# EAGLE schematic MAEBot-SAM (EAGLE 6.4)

## Sheet 1 of 4: SAMA5
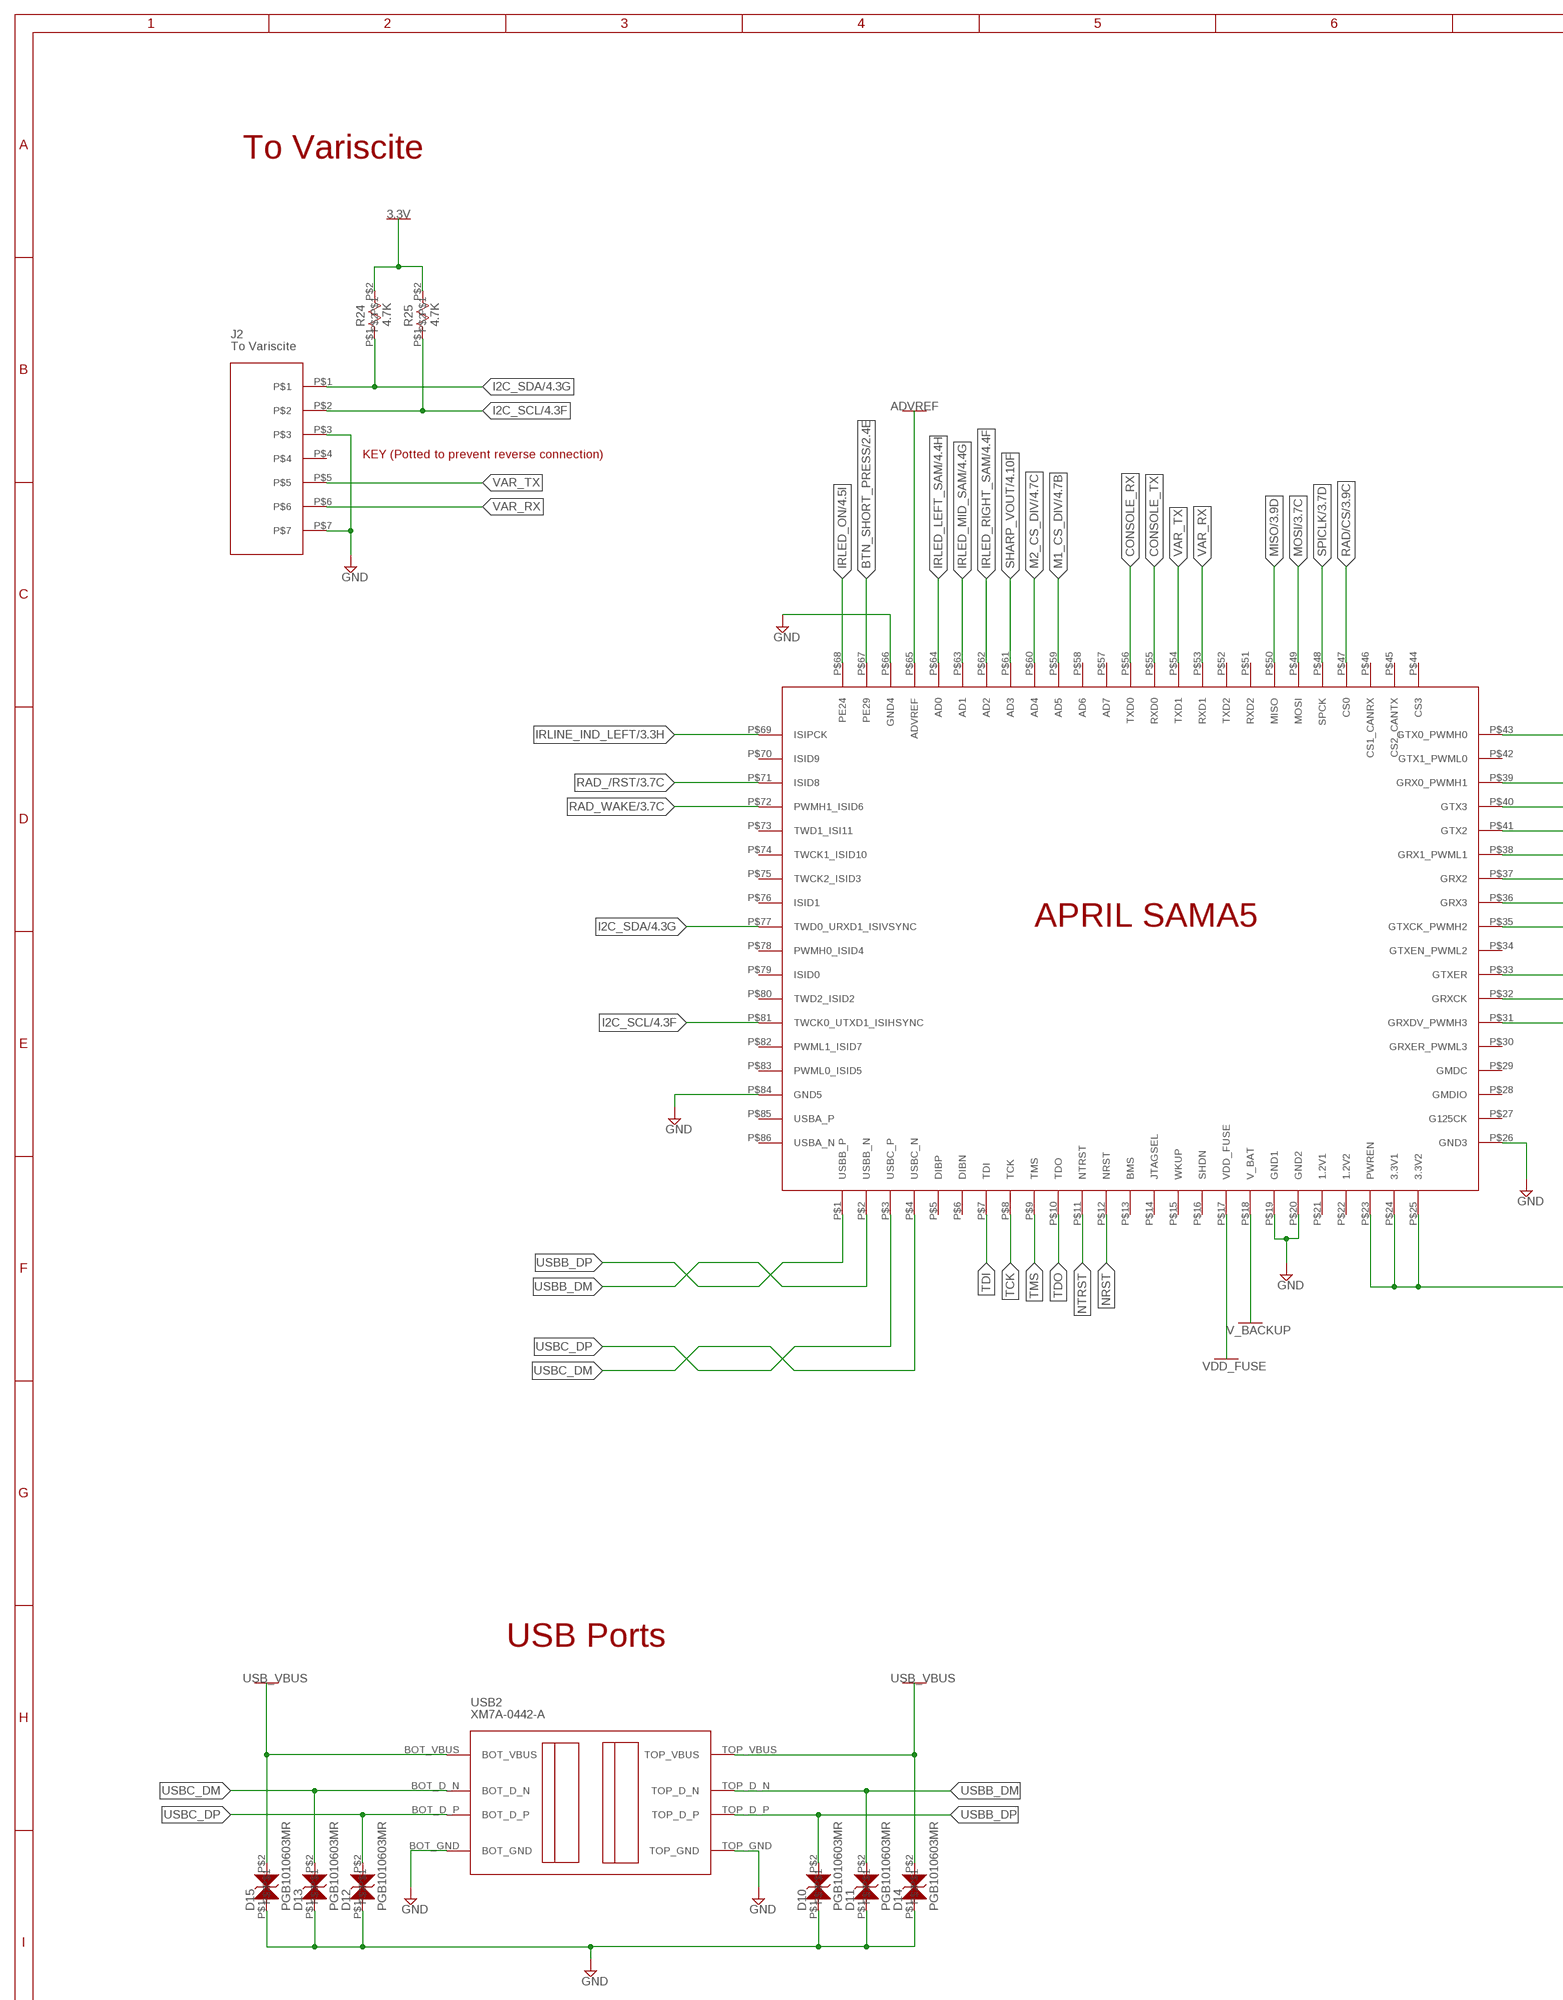
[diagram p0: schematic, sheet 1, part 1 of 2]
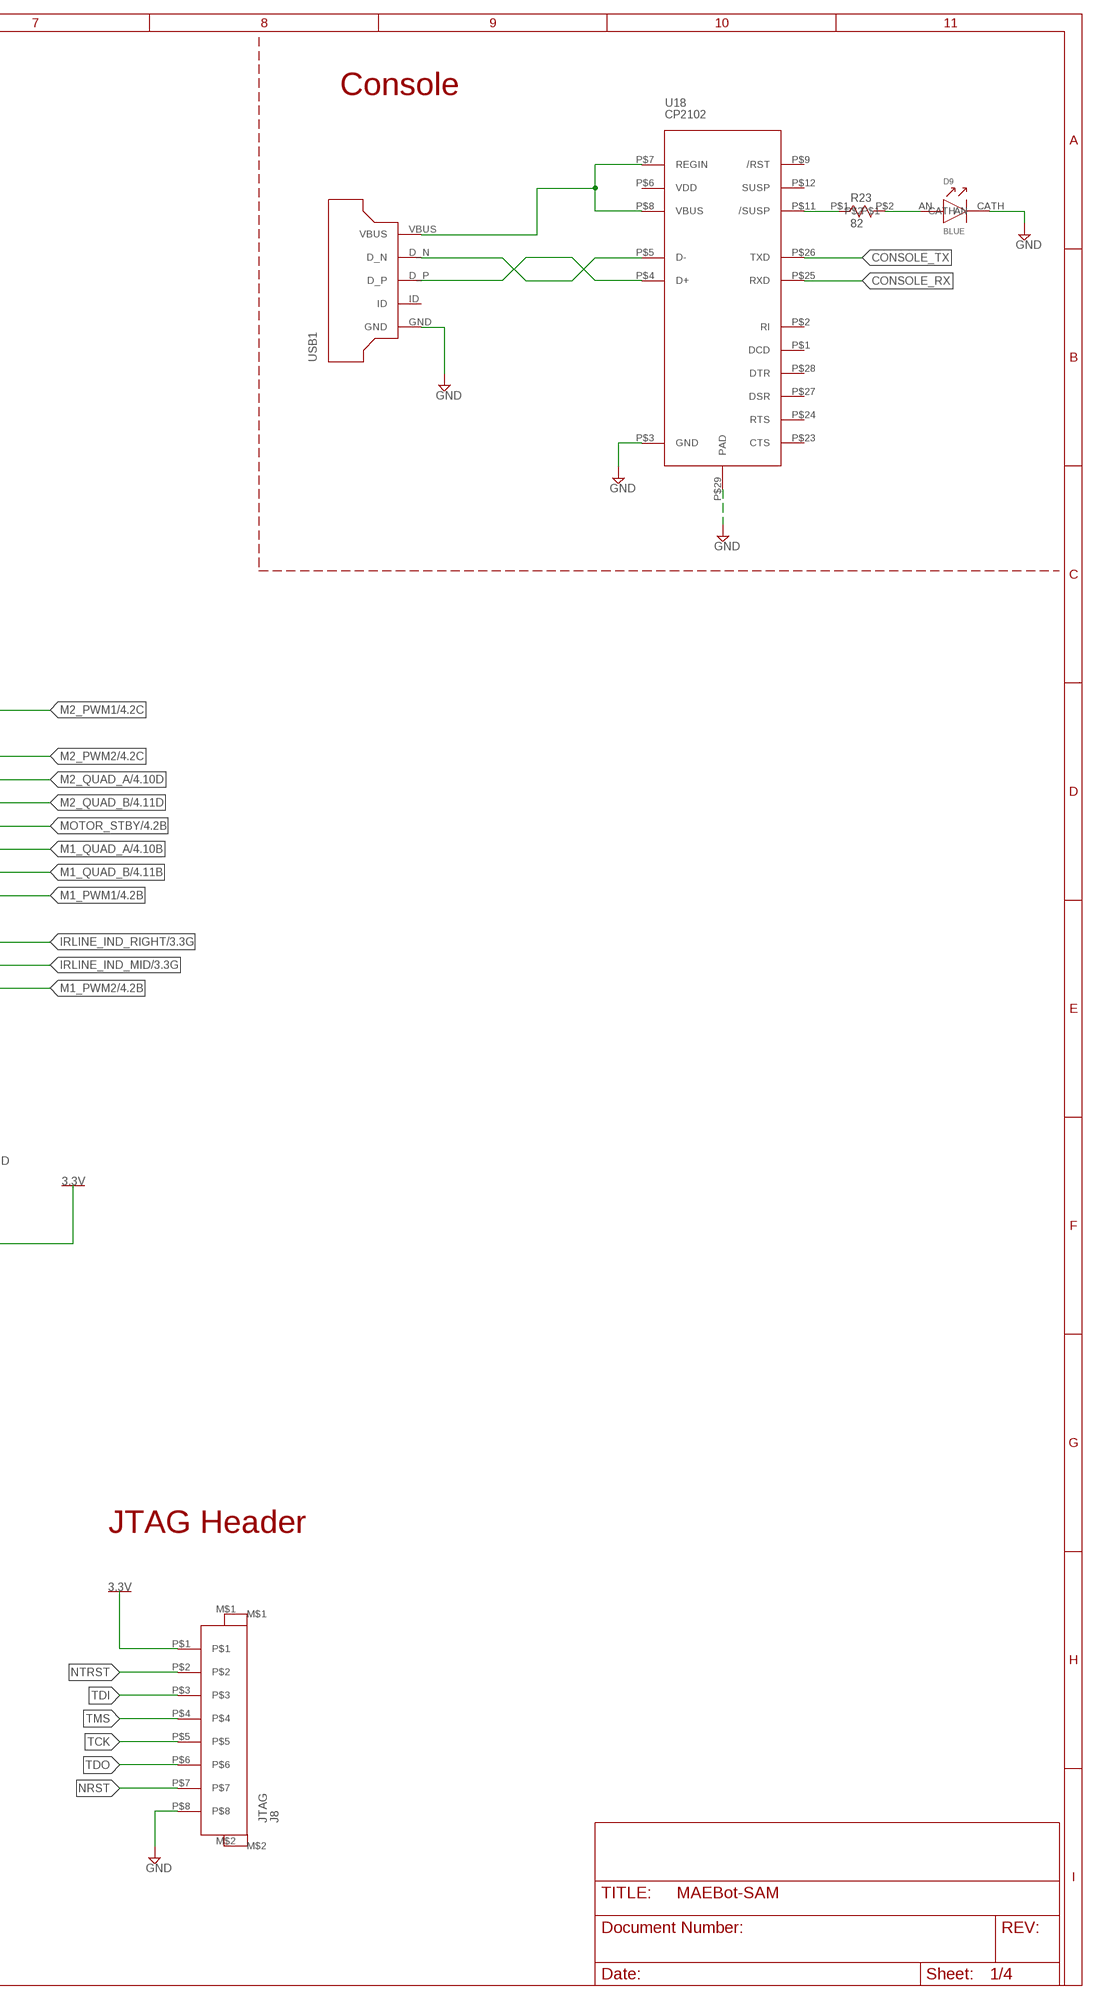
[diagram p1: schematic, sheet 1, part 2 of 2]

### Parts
D9  BLUE  LED0603  [D0603]
D10  PGB1010603MR  TVS0603  [SM0603]
D11  PGB1010603MR  TVS0603  [SM0603]
D12  PGB1010603MR  TVS0603  [SM0603]
D13  PGB1010603MR  TVS0603  [SM0603]
D14  PGB1010603MR  TVS0603  [SM0603]
D15  PGB1010603MR  TVS0603  [SM0603]
J2  To Variscite  J7X1  [J7X1]
J8  JTAG  PICOBLADE-8  [PICO-8]
R23  82  R0402  [R0402]
R24  4.7K  R0402  [R0402]
R25  4.7K  R0402  [R0402]
SAMA1  SAMA5_CARRIER  [SAMA5_CARRIER]
U18  CP2102  [28QFN-5MM]
USB1  USB_MINI_A  [USB_MINI_A]
USB2  XM7A-0442-A  [XM7A-0442-A]

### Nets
3.3V: J8.P$1 R24.P$2 R25.P$2 SAMA1.P$23(PWREN) SAMA1.P$24(3.3V1) SAMA1.P$25(3.3V2) ; also sheet 2,3,4
ADVREF: SAMA1.P$65(ADVREF) ; also sheet 2,4
BTN_SHORT_PRESS: SAMA1.P$67(PE29) ; also sheet 2,3
CONSOLE_/SUSP: R23.P$1 U18.P$11(/SUSP)
CONSOLE_DM: U18.P$5(D-) USB1.D_N
CONSOLE_DP: U18.P$4(D+) USB1.D_P
CONSOLE_LED: D9.AN R23.P$2
CONSOLE_RX: SAMA1.P$56(TXD0) U18.P$25(RXD)
CONSOLE_TX: SAMA1.P$55(RXD0) U18.P$26(TXD)
CONSOLE_VBUS: U18.P$7(REGIN) U18.P$8(VBUS) USB1.VBUS
GND: D9.CATH D10.P$1 D11.P$1 D12.P$1 D13.P$1 D14.P$1 D15.P$1 J2.P$3 J2.P$7 J8.P$8 SAMA1.P$19(GND1) SAMA1.P$20(GND2) SAMA1.P$26(GND3) SAMA1.P$66(GND4) SAMA1.P$84(GND5) U18.P$3(GND) U18.P$29(PAD) USB1.GND USB2.BOT_GND USB2.TOP_GND ; also sheet 2,3,4
I2C_SCL: J2.P$2 R25.P$1 SAMA1.P$81(TWCK0_UTXD1_ISIHSYNC) ; also sheet 4
I2C_SDA: J2.P$1 R24.P$1 SAMA1.P$77(TWD0_URXD1_ISIVSYNC) ; also sheet 4
IRLED_LEFT_SAM: SAMA1.P$64(AD0) ; also sheet 4
IRLED_MID_SAM: SAMA1.P$63(AD1) ; also sheet 4
IRLED_ON: SAMA1.P$68(PE24) ; also sheet 4
IRLED_RIGHT_SAM: SAMA1.P$62(AD2) ; also sheet 4
IRLINE_IND_LEFT: SAMA1.P$69(ISIPCK) ; also sheet 3
IRLINE_IND_MID: SAMA1.P$32(GRXCK) ; also sheet 3
IRLINE_IND_RIGHT: SAMA1.P$33(GTXER) ; also sheet 3
M1_CS_DIV: SAMA1.P$59(AD5) ; also sheet 4
M1_PWM1: SAMA1.P$35(GTXCK_PWMH2) ; also sheet 4
M1_PWM2: SAMA1.P$31(GRXDV_PWMH3) ; also sheet 4
M1_QUAD_A: SAMA1.P$37(GRX2) ; also sheet 4
M1_QUAD_B: SAMA1.P$36(GRX3) ; also sheet 4
M2_CS_DIV: SAMA1.P$60(AD4) ; also sheet 4
M2_PWM1: SAMA1.P$43(GTX0_PWMH0) ; also sheet 4
M2_PWM2: SAMA1.P$39(GRX0_PWMH1) ; also sheet 4
M2_QUAD_A: SAMA1.P$40(GTX3) ; also sheet 4
M2_QUAD_B: SAMA1.P$41(GTX2) ; also sheet 4
MISO: SAMA1.P$50(MISO) ; also sheet 3
MOSI: SAMA1.P$49(MOSI) ; also sheet 3
MOTOR_STBY: SAMA1.P$38(GRX1_PWML1) ; also sheet 4
NRST: J8.P$7 SAMA1.P$12(NRST)
NTRST: J8.P$2 SAMA1.P$11(NTRST)
RAD/CS: SAMA1.P$47(CS0) ; also sheet 3
RAD_/RST: SAMA1.P$71(ISID8) ; also sheet 3
RAD_WAKE: SAMA1.P$72(PWMH1_ISID6) ; also sheet 3
SHARP_VOUT: SAMA1.P$61(AD3) ; also sheet 4
SPICLK: SAMA1.P$48(SPCK) ; also sheet 3
TCK: J8.P$5 SAMA1.P$8(TCK)
TDI: J8.P$3 SAMA1.P$7(TDI)
TDO: J8.P$6 SAMA1.P$10(TDO)
TMS: J8.P$4 SAMA1.P$9(TMS)
USB_VBUS: D14.P$2 D15.P$2 USB2.BOT_VBUS USB2.TOP_VBUS ; also sheet 2
USBB_DM: D11.P$2 SAMA1.P$2(USBB_N) USB2.TOP_D_N
USBB_DP: D10.P$2 SAMA1.P$1(USBB_P) USB2.TOP_D_P
USBC_DM: D13.P$2 SAMA1.P$4(USBC_N) USB2.BOT_D_N
USBC_DP: D12.P$2 SAMA1.P$3(USBC_P) USB2.BOT_D_P
V_BACKUP: SAMA1.P$18(V_BAT) ; also sheet 2,3
VAR_RX: J2.P$6 SAMA1.P$53(RXD1)
VAR_TX: J2.P$5 SAMA1.P$54(TXD1)
VDD_FUSE: SAMA1.P$17(VDD_FUSE) ; also sheet 2
Unconnected: J2.P$4 J8.M$1 J8.M$2 SAMA1.P$5(DIBP) SAMA1.P$6(DIBN) SAMA1.P$13(BMS) SAMA1.P$14(JTAGSEL) SAMA1.P$15(WKUP) SAMA1.P$16(SHDN) SAMA1.P$21(1.2V1) SAMA1.P$22(1.2V2) SAMA1.P$27(G125CK) SAMA1.P$28(GMDIO) SAMA1.P$29(GMDC) SAMA1.P$30(GRXER_PWML3) SAMA1.P$34(GTXEN_PWML2) SAMA1.P$42(GTX1_PWML0) SAMA1.P$44(CS3) SAMA1.P$45(CS2_CANTX) SAMA1.P$46(CS1_CANRX) SAMA1.P$51(RXD2) SAMA1.P$52(TXD2) SAMA1.P$57(AD7) SAMA1.P$58(AD6) SAMA1.P$70(ISID9) SAMA1.P$73(TWD1_ISI11) SAMA1.P$74(TWCK1_ISID10) SAMA1.P$75(TWCK2_ISID3) SAMA1.P$76(ISID1) SAMA1.P$78(PWMH0_ISID4) SAMA1.P$79(ISID0) SAMA1.P$80(TWD2_ISID2) SAMA1.P$82(PWML1_ISID7) SAMA1.P$83(PWML0_ISID5) SAMA1.P$85(USBA_P) SAMA1.P$86(USBA_N) U18.P$1(DCD) U18.P$2(RI) U18.P$9(/RST) U18.P$12(SUSP) U18.P$23(CTS) U18.P$24(RTS) U18.P$27(DSR) U18.P$28(DTR) USB1.ID

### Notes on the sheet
- Console
- To Variscite
- KEY (Potted to prevent reverse connection)
- APRIL SAMA5
- JTAG Header
- USB Ports

## Sheet 2 of 4: Power
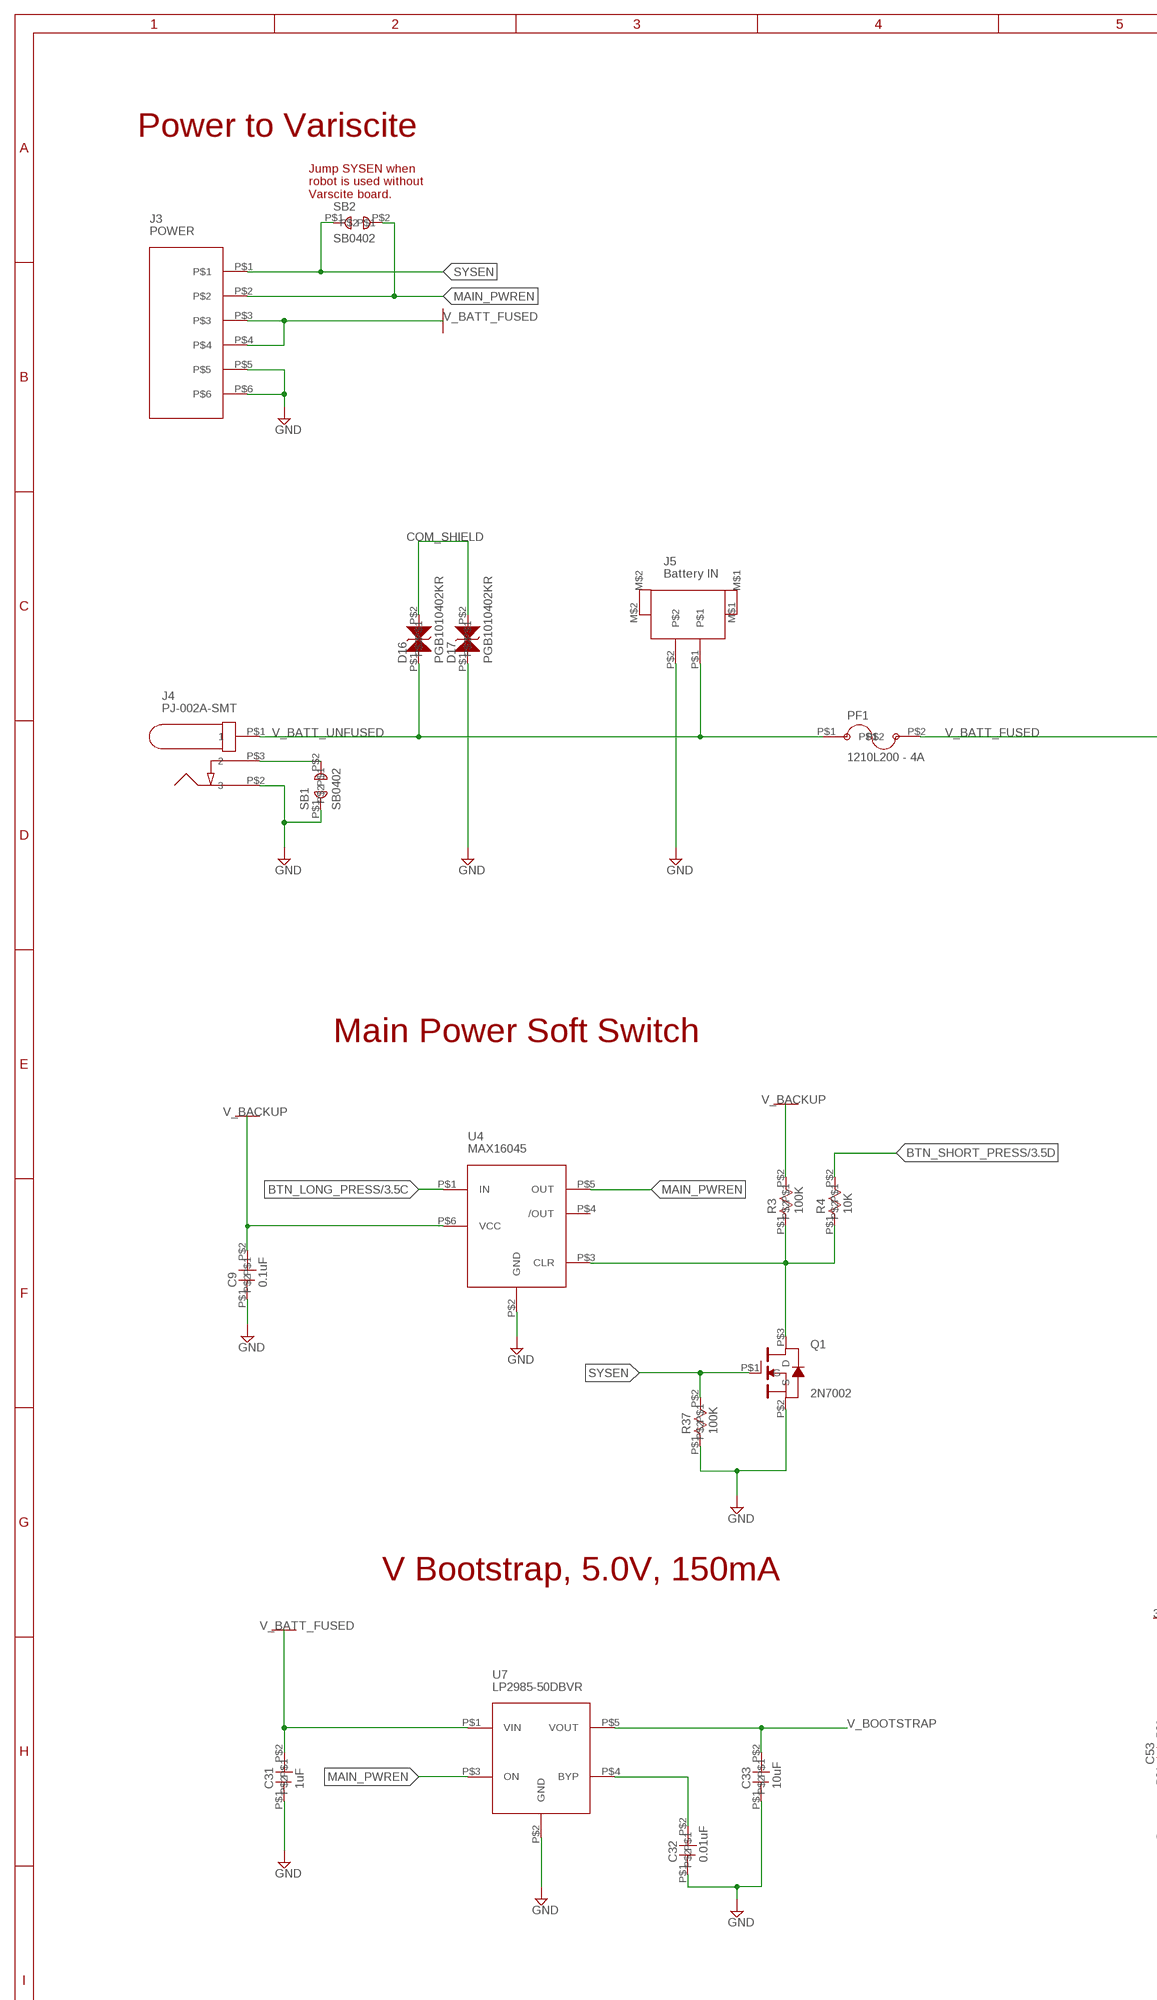
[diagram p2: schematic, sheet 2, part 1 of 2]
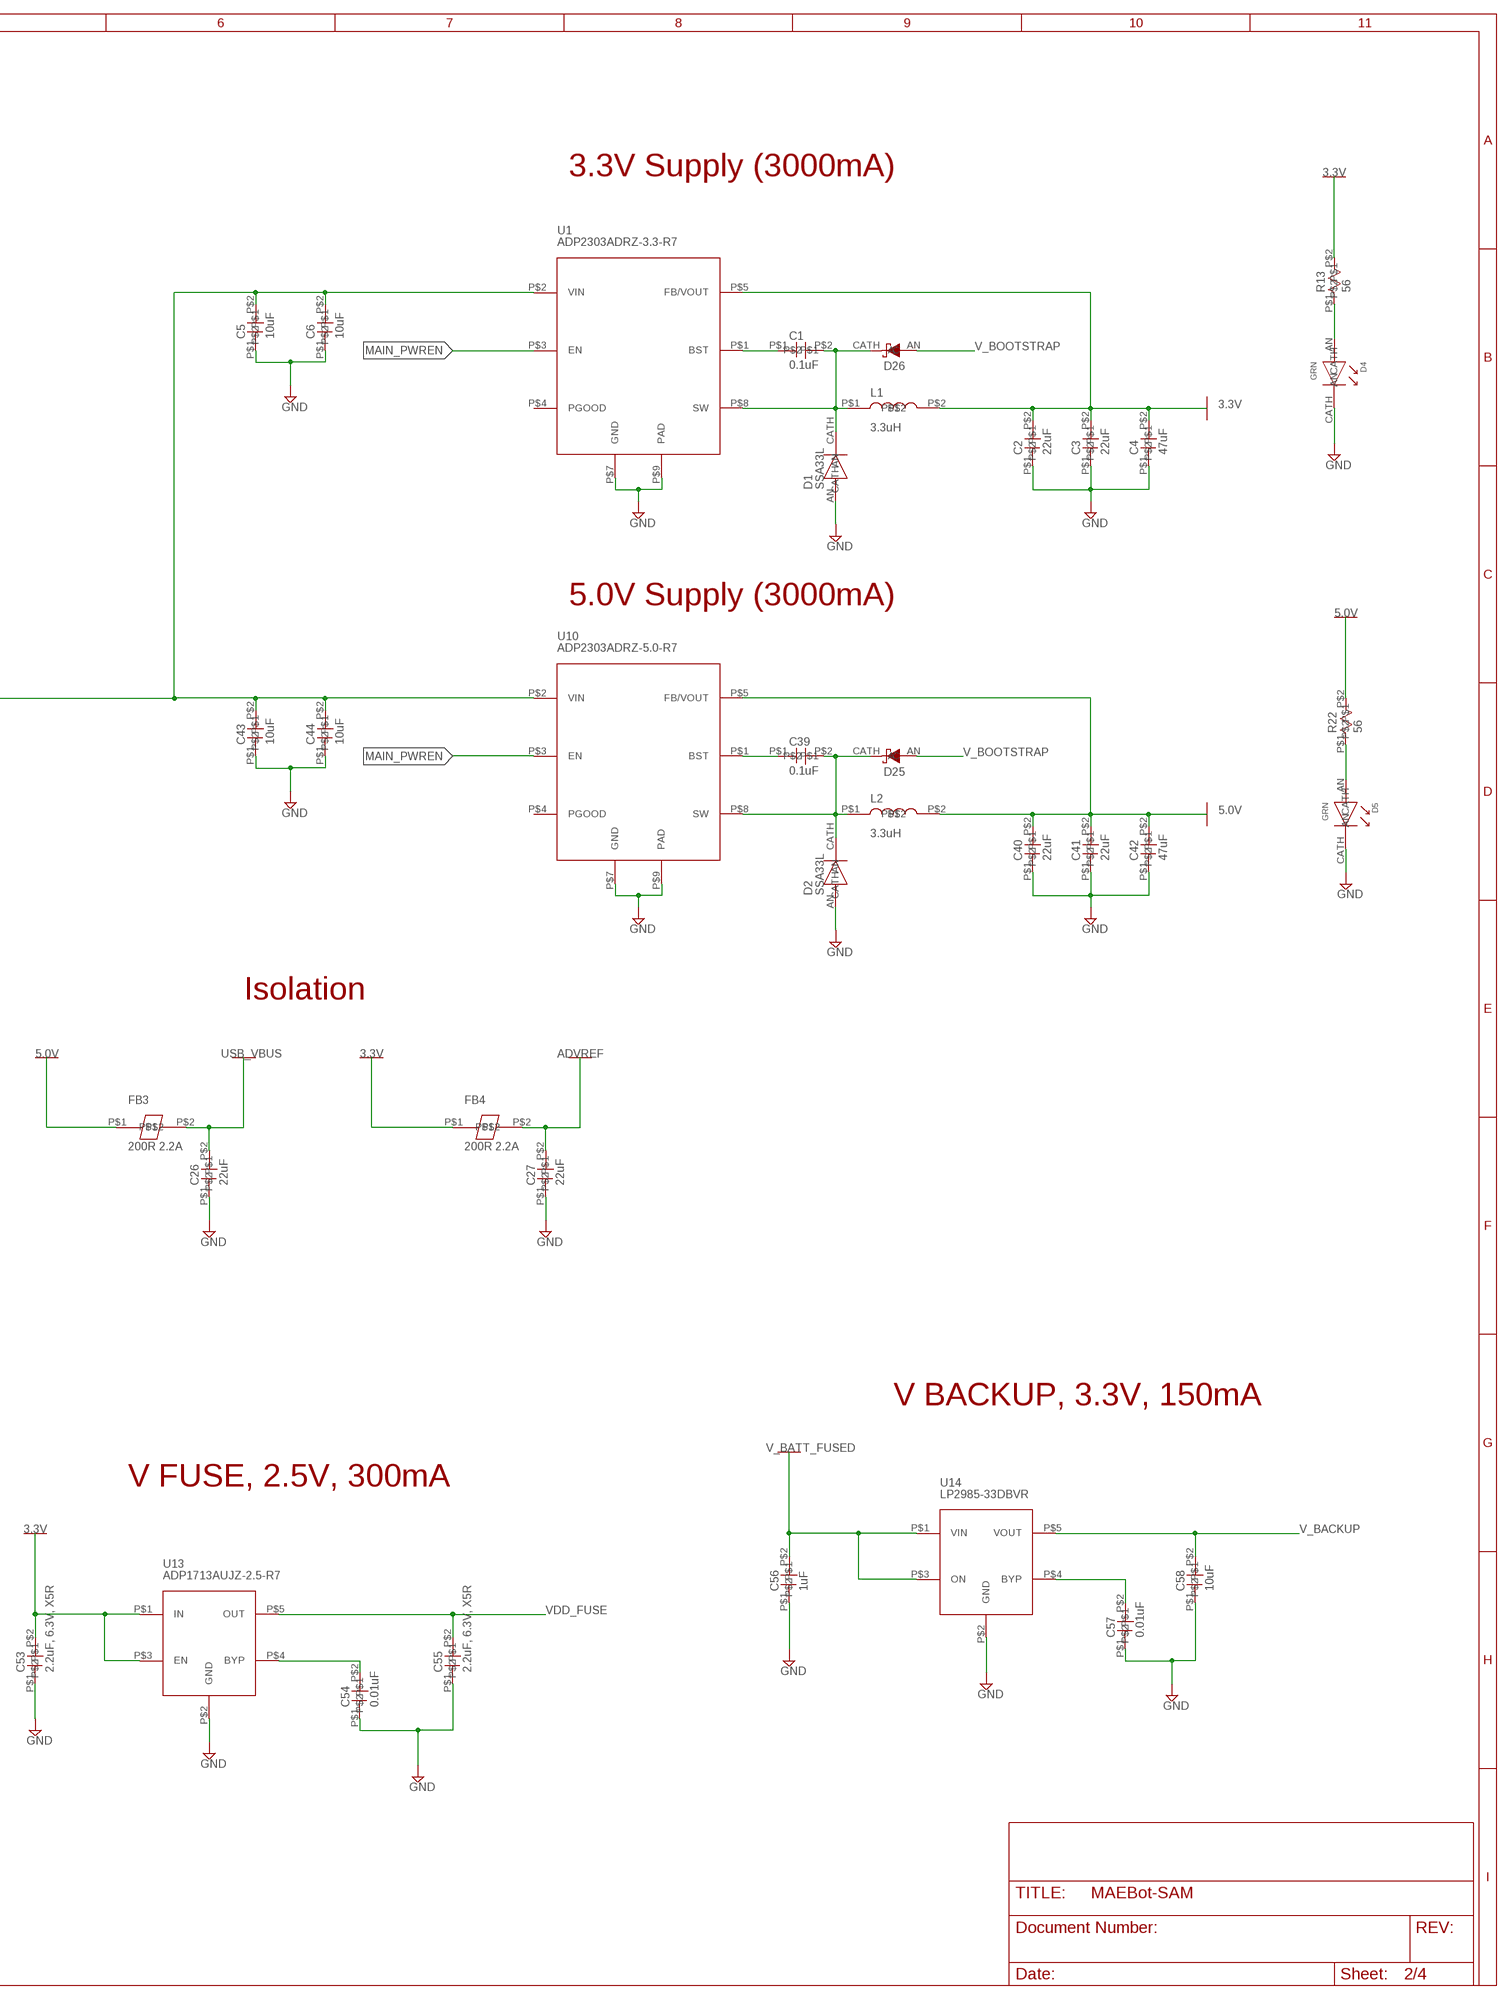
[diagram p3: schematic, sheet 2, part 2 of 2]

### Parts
C1  0.1uF  C0402  [R0402]
C2  22uF  C0603  [SM0603]
C3  22uF  C0603  [SM0603]
C4  47uF  C0805  [SM0805]
C5  10uF  C0603  [SM0603]
C6  10uF  C0603  [SM0603]
C9  0.1uF  C0402  [R0402]
C26  22uF  C0603  [SM0603]
C27  22uF  C0603  [SM0603]
C31  1uF  C0402  [R0402]
C32  0.01uF  C0402  [R0402]
C33  10uF  C0805  [SM0805]
C39  0.1uF  C0402  [R0402]
C40  22uF  C0603  [SM0603]
C41  22uF  C0603  [SM0603]
C42  47uF  C0805  [SM0805]
C43  10uF  C0603  [SM0603]
C44  10uF  C0603  [SM0603]
C53  2.2uF, 6.3V, X5R  C0402  [R0402]
C54  0.01uF  C0402  [R0402]
C55  2.2uF, 6.3V, X5R  C0805  [SM0805]
C56  1uF  C0402  [R0402]
C57  0.01uF  C0402  [R0402]
C58  10uF  C0805  [SM0805]
D1  SSA33L  [SSA33L]
D2  SSA33L  [SSA33L]
D4  GRN  LED0603  [D0603]
D5  GRN  LED0603  [D0603]
D16  PGB1010402KR  TVS0402  [R0402]
D17  PGB1010402KR  TVS0402  [R0402]
D25  DS0603  [D0603]
D26  DS0603  [D0603]
FB3  200R 2.2A  FB0603  [SM0603]
FB4  200R 2.2A  FB0603  [SM0603]
J3  POWER  J6X1  [J6X1]
J4  PJ-002A-SMT  [PJ-002A-SMT]
J5  Battery IN  PICOBLADE-2  [PICO-2]
L1  3.3uH  VLF10040  [VLF10040_SERIES]
L2  3.3uH  VLF10040  [VLF10040_SERIES]
PF1  1210L200 - 4A  1210L  [1210L_SERIES]
Q1  2N7002  [SOT23]
R3  100K  R0402  [R0402]
R4  10K  R0402  [R0402]
R13  56  R0402  [R0402]
R22  56  R0402  [R0402]
R37  100K  R0402  [R0402]
SB1  SB0402  [R0402]
SB2  SB0402  [R0402]
U1  ADP2303ADRZ-3.3-R7  [RD-8-1]
U4  MAX16045  [90-0240]
U7  LP2985-50DBVR  LP2985  [R-PDS0-G5_(SOT23-5)]
U10  ADP2303ADRZ-5.0-R7  [RD-8-1]
U13  ADP1713AUJZ-2.5-R7  ADP1713  [ADP171X_(SOT23-5)]
U14  LP2985-33DBVR  LP2985  [R-PDS0-G5_(SOT23-5)]

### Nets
3.3V: C2.P$2 C3.P$2 C4.P$2 C53.P$2 FB4.P$1 L1.P$2 R13.P$2 U1.P$5(FB/VOUT) U13.P$1(IN) U13.P$3(EN) ; also sheet 1,3,4
3.3V_BYP: C57.P$2 U14.P$4(BYP)
5.0V: C40.P$2 C41.P$2 C42.P$2 FB3.P$1 L2.P$2 R22.P$2 U10.P$5(FB/VOUT) ; also sheet 4
5.0V_BYP: C32.P$2 U7.P$4(BYP)
ADVREF: C27.P$2 FB4.P$2 ; also sheet 1,4
BST: C1.P$1 U1.P$1(BST)
BST1: C39.P$1 U10.P$1(BST)
BTN_LONG_PRESS: U4.P$1(IN) ; also sheet 3
BTN_SHORT_PRESS: R4.P$2 ; also sheet 1,3
CHG_GND2: J4.P$3 SB1.P$2
COM_SHIELD: D16.P$2 D17.P$2
GND: C2.P$1 C3.P$1 C4.P$1 C5.P$1 C6.P$1 C9.P$1 C26.P$1 C27.P$1 C31.P$1 C32.P$1 C33.P$1 C40.P$1 C41.P$1 C42.P$1 C43.P$1 C44.P$1 C53.P$1 C54.P$1 C55.P$1 C56.P$1 C57.P$1 C58.P$1 D1.AN D2.AN D4.CATH D5.CATH D17.P$1 J3.P$5 J3.P$6 J4.P$2 J5.P$2 Q1.P$2(S) R37.P$1 SB1.P$1 U1.P$7(GND) U1.P$9(PAD) U4.P$2(GND) U7.P$2(GND) U10.P$7(GND) U10.P$9(PAD) U13.P$2(GND) U14.P$2(GND) ; also sheet 1,3,4
IND_3.3V: D4.AN R13.P$1
IND_5.0V: D5.AN R22.P$1
MAIN_PWREN: J3.P$2 SB2.P$2 U1.P$3(EN) U4.P$5(OUT) U7.P$3(ON) U10.P$3(EN)
N$66: C54.P$2 U13.P$4(BYP)
SOFTPWR_CLR: Q1.P$3(D) R3.P$1 R4.P$1 U4.P$3(CLR)
SW_3.3V: C1.P$2 D1.CATH D26.CATH(C) L1.P$1 U1.P$8(SW)
SW_5V: C39.P$2 D2.CATH D25.CATH(C) L2.P$1 U10.P$8(SW)
SYSEN: J3.P$1 Q1.P$1(G) R37.P$2 SB2.P$1
USB_VBUS: C26.P$2 FB3.P$2 ; also sheet 1
V_BACKUP: C9.P$2 C58.P$2 R3.P$2 U4.P$6(VCC) U14.P$5(VOUT) ; also sheet 1,3
V_BATT_FUSED: C5.P$2 C6.P$2 C31.P$2 C43.P$2 C44.P$2 C56.P$2 J3.P$3 J3.P$4 PF1.P$2 U1.P$2(VIN) U7.P$1(VIN) U10.P$2(VIN) U14.P$1(VIN) U14.P$3(ON)
V_BATT_UNFUSED: D16.P$1 J4.P$1 J5.P$1 PF1.P$1
V_BOOTSTRAP: C33.P$2 D25.AN(A) D26.AN(A) U7.P$5(VOUT)
VDD_FUSE: C55.P$2 U13.P$5(OUT) ; also sheet 1
Unconnected: J5.M$1 J5.M$2 U1.P$4(PGOOD) U4.P$4(/OUT) U10.P$4(PGOOD)

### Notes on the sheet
- Power to Variscite
- 3.3V Supply (3000mA)
- Jump SYSEN when
  robot is used without 
  Varscite board.
- 5.0V Supply (3000mA)
- Main Power Soft Switch
- Isolation
- V BACKUP, 3.3V, 150mA
- V FUSE, 2.5V, 300mA
- V Bootstrap, 5.0V, 150mA

## Sheet 3 of 4: UI
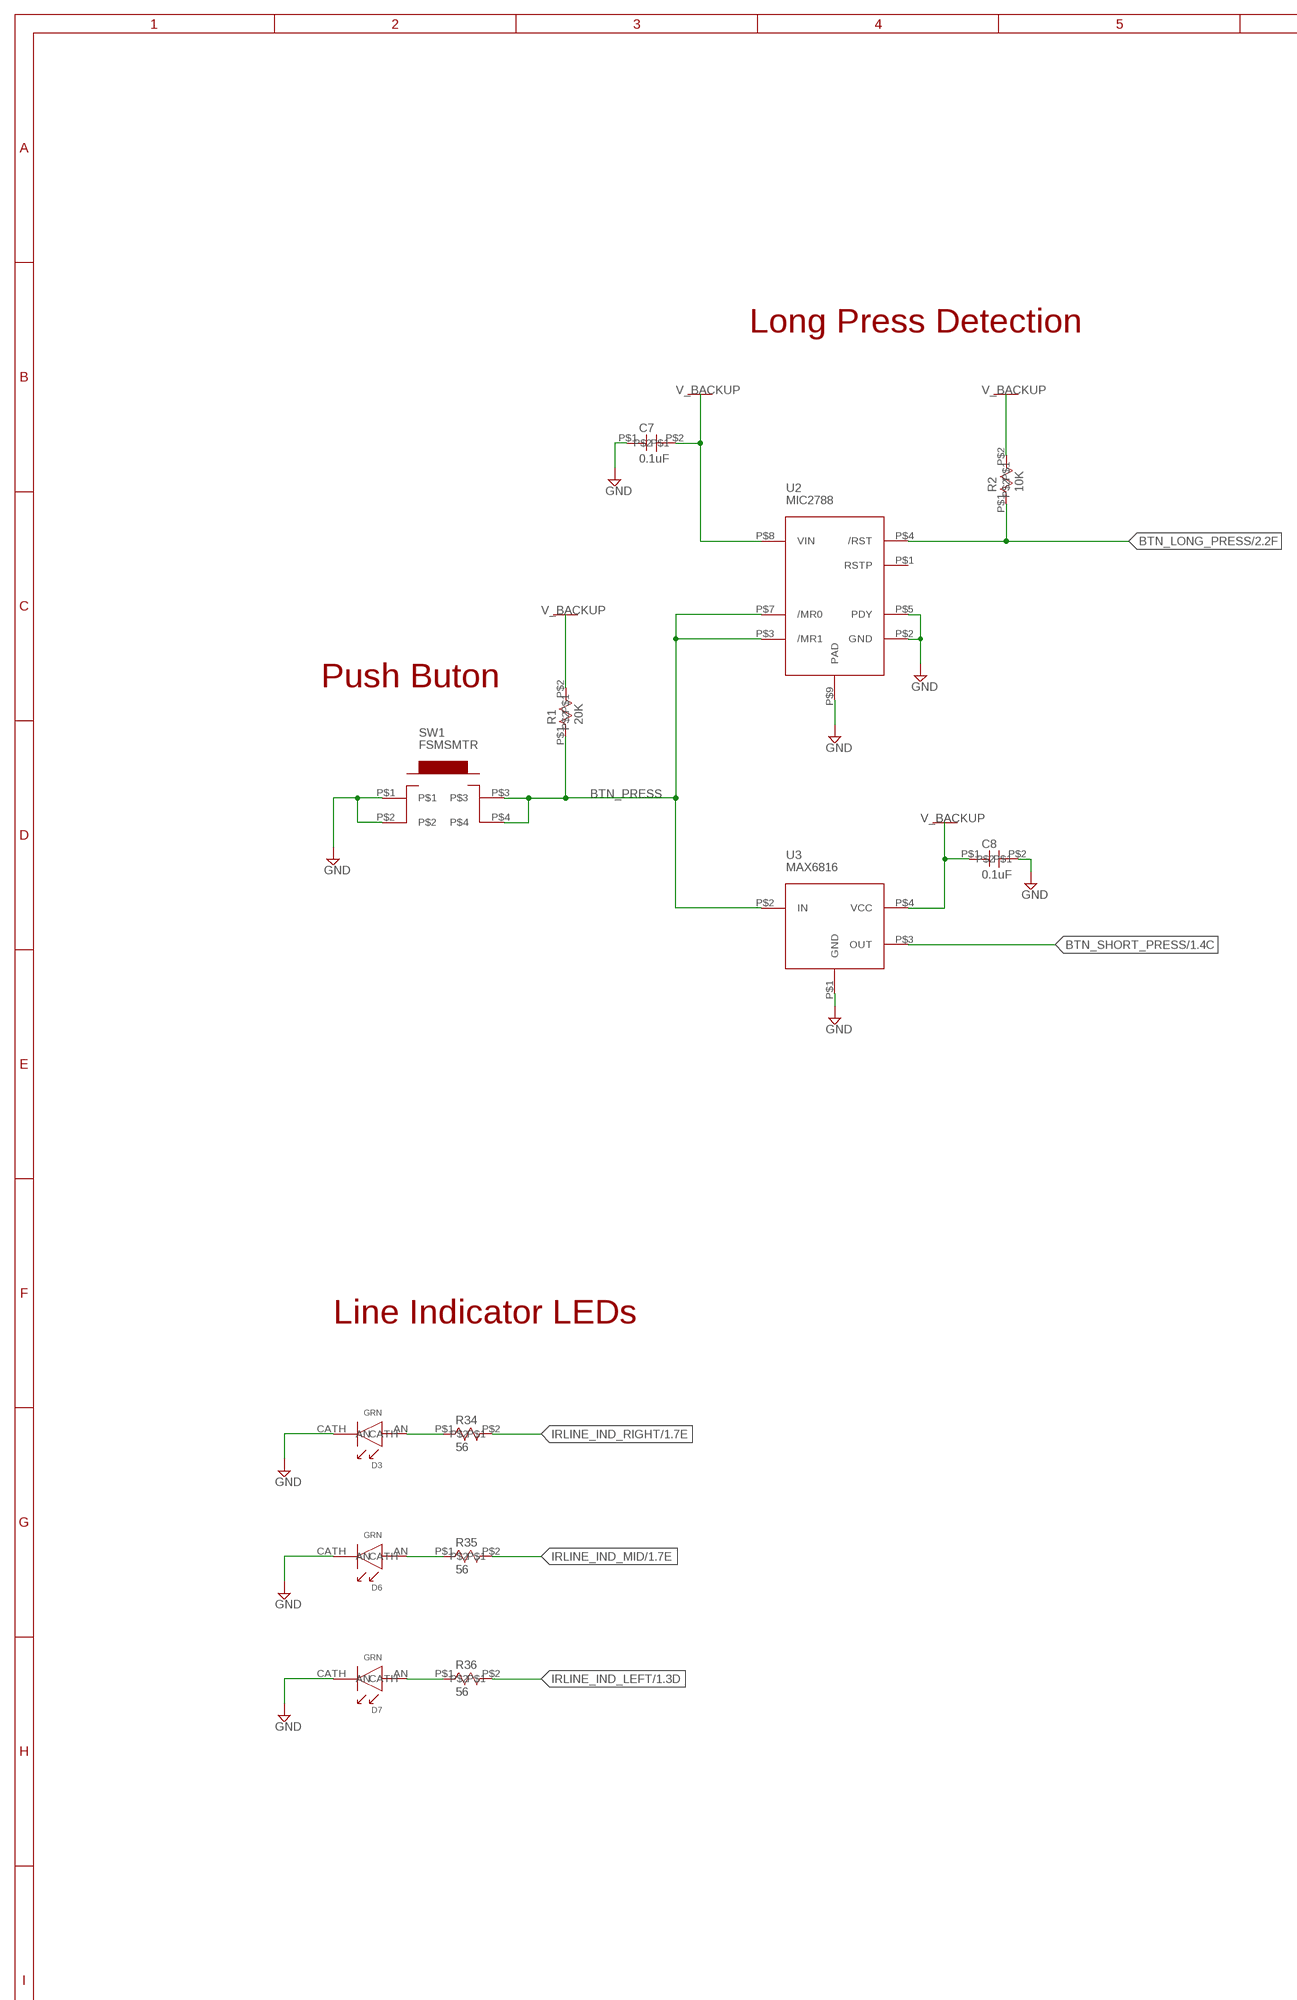
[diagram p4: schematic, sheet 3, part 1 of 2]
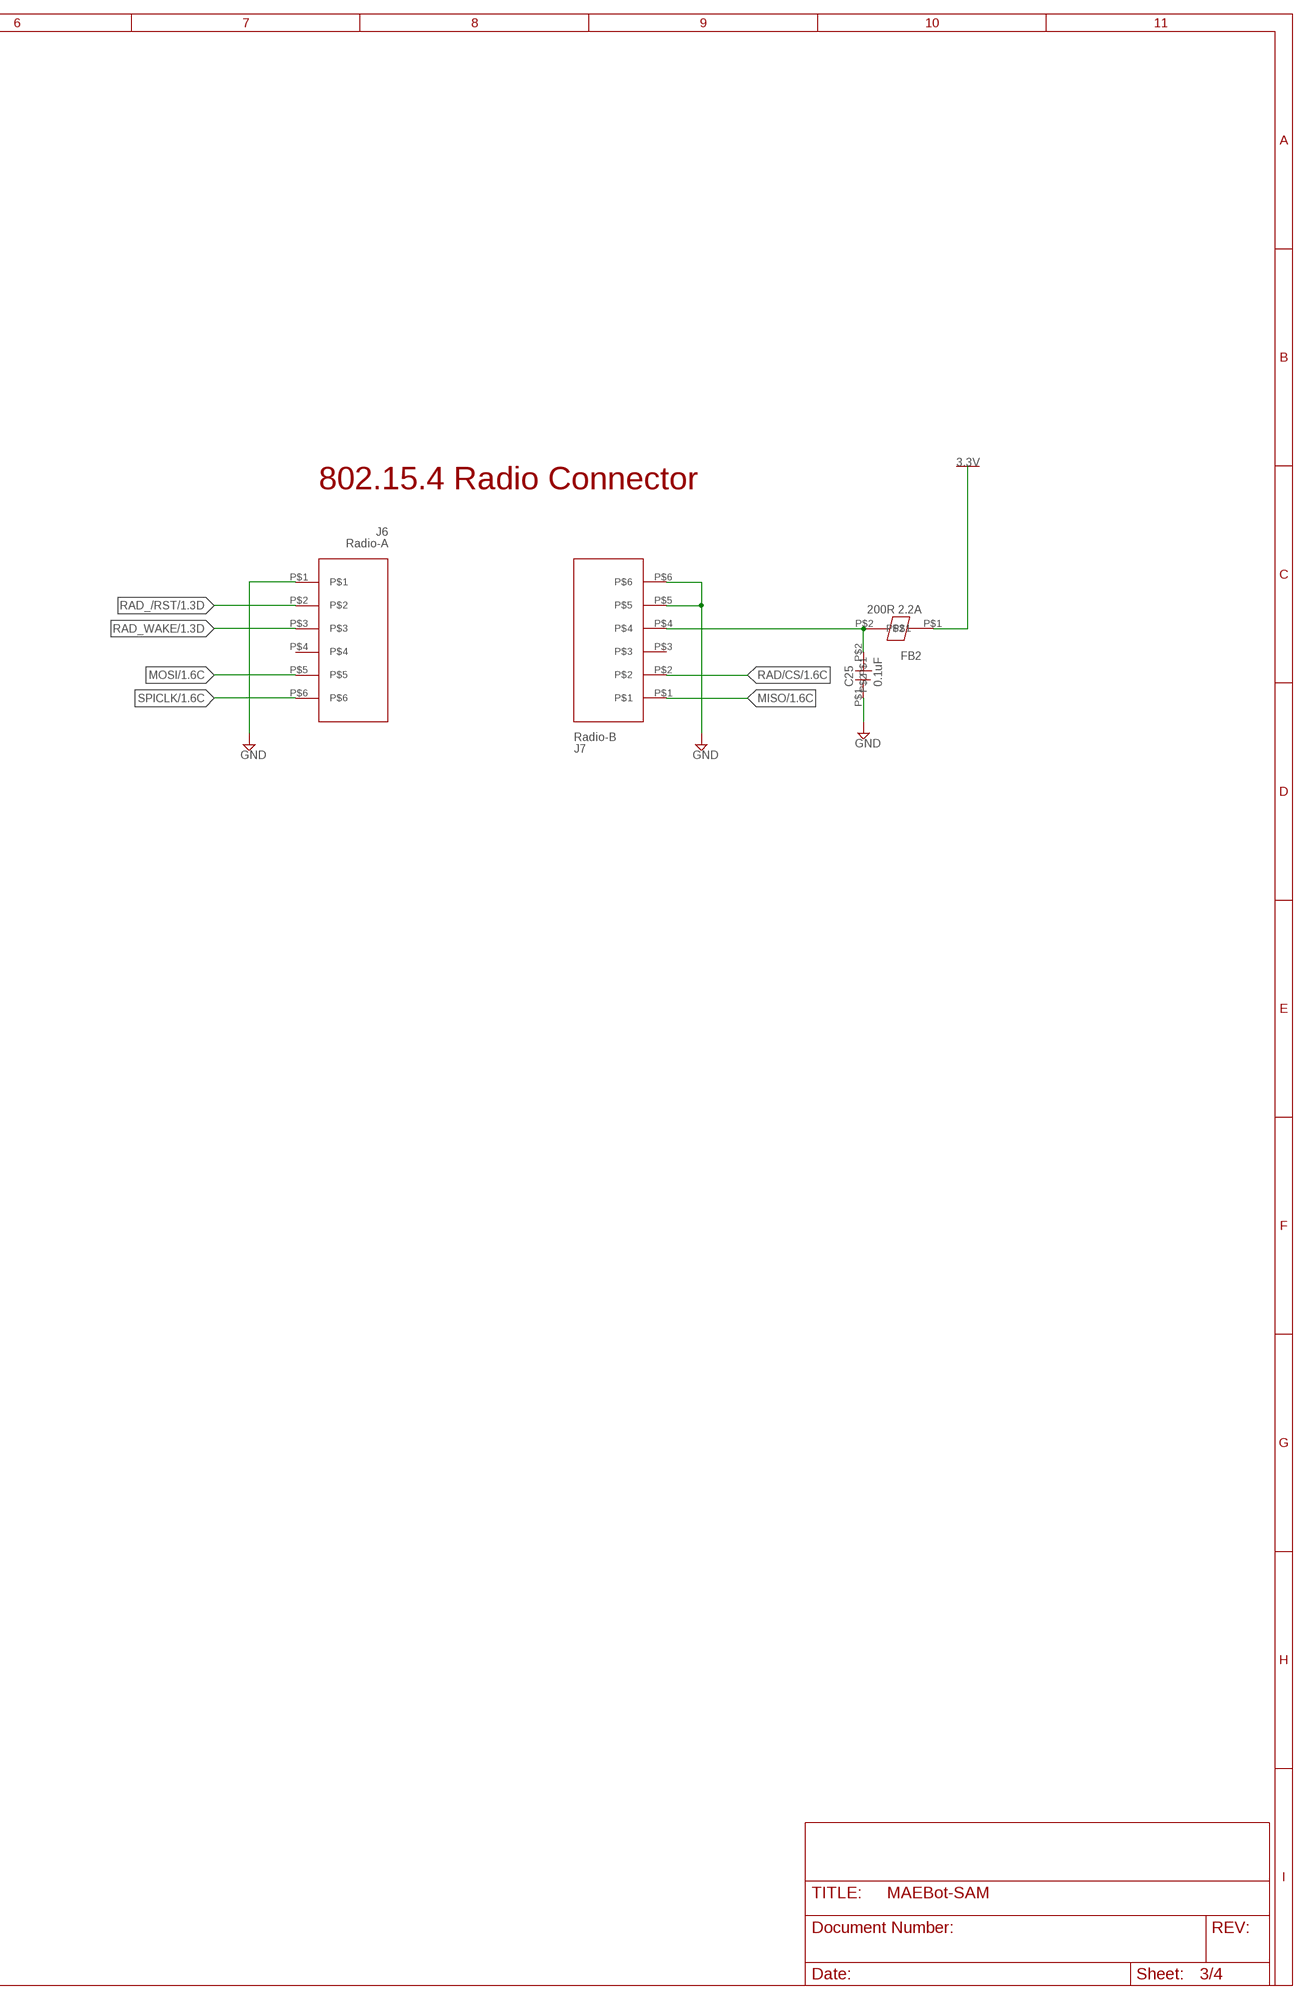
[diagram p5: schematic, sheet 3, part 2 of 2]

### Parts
C7  0.1uF  C0402  [R0402]
C8  0.1uF  C0402  [R0402]
C25  0.1uF  C0402  [R0402]
D3  GRN  LED0603  [D0603]
D6  GRN  LED0603  [D0603]
D7  GRN  LED0603  [D0603]
FB2  200R 2.2A  FB0603  [SM0603]
J6  Radio-A  J6X1  [J6X1]
J7  Radio-B  J6X1  [J6X1]
R1  20K  R0402  [R0402]
R2  10K  R0402  [R0402]
R34  56  R0402  [R0402]
R35  56  R0402  [R0402]
R36  56  R0402  [R0402]
SW1  FSMSMTR  FSMJSMA  [FSMJSMA]
U2  MIC2788  [MLF8]
U3  MAX6816  [90-0183]

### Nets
3.3V: FB2.P$1 ; also sheet 1,2,4
BTN_LONG_PRESS: R2.P$1 U2.P$4(/RST) ; also sheet 2
BTN_PRESS: R1.P$1 SW1.P$3 SW1.P$4 U2.P$3(/MR1) U2.P$7(/MR0) U3.P$2(IN)
BTN_SHORT_PRESS: U3.P$3(OUT) ; also sheet 1,2
GND: C7.P$1 C8.P$2 C25.P$1 D3.CATH D6.CATH D7.CATH J6.P$1 J7.P$5 J7.P$6 SW1.P$1 SW1.P$2 U2.P$2(GND) U2.P$5(PDY) U2.P$9(PAD) U3.P$1(GND) ; also sheet 1,2,4
IRLINE_IND_LEFT: R36.P$2 ; also sheet 1
IRLINE_IND_MID: R35.P$2 ; also sheet 1
IRLINE_IND_RIGHT: R34.P$2 ; also sheet 1
MISO: J7.P$1 ; also sheet 1
MOSI: J6.P$5 ; also sheet 1
N$1: D3.AN R34.P$1
N$4: D6.AN R35.P$1
N$5: D7.AN R36.P$1
RAD/CS: J7.P$2 ; also sheet 1
RAD_/RST: J6.P$2 ; also sheet 1
RAD_VIN: C25.P$2 FB2.P$2 J7.P$4
RAD_WAKE: J6.P$3 ; also sheet 1
SPICLK: J6.P$6 ; also sheet 1
V_BACKUP: C7.P$2 C8.P$1 R1.P$2 R2.P$2 U2.P$8(VIN) U3.P$4(VCC) ; also sheet 1,2
Unconnected: J6.P$4 J7.P$3 U2.P$1(RSTP)

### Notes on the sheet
- Long Press Detection
- 802.15.4 Radio Connector
- Push Buton
- Line Indicator LEDs

## Sheet 4 of 4: Sensors and Actuators
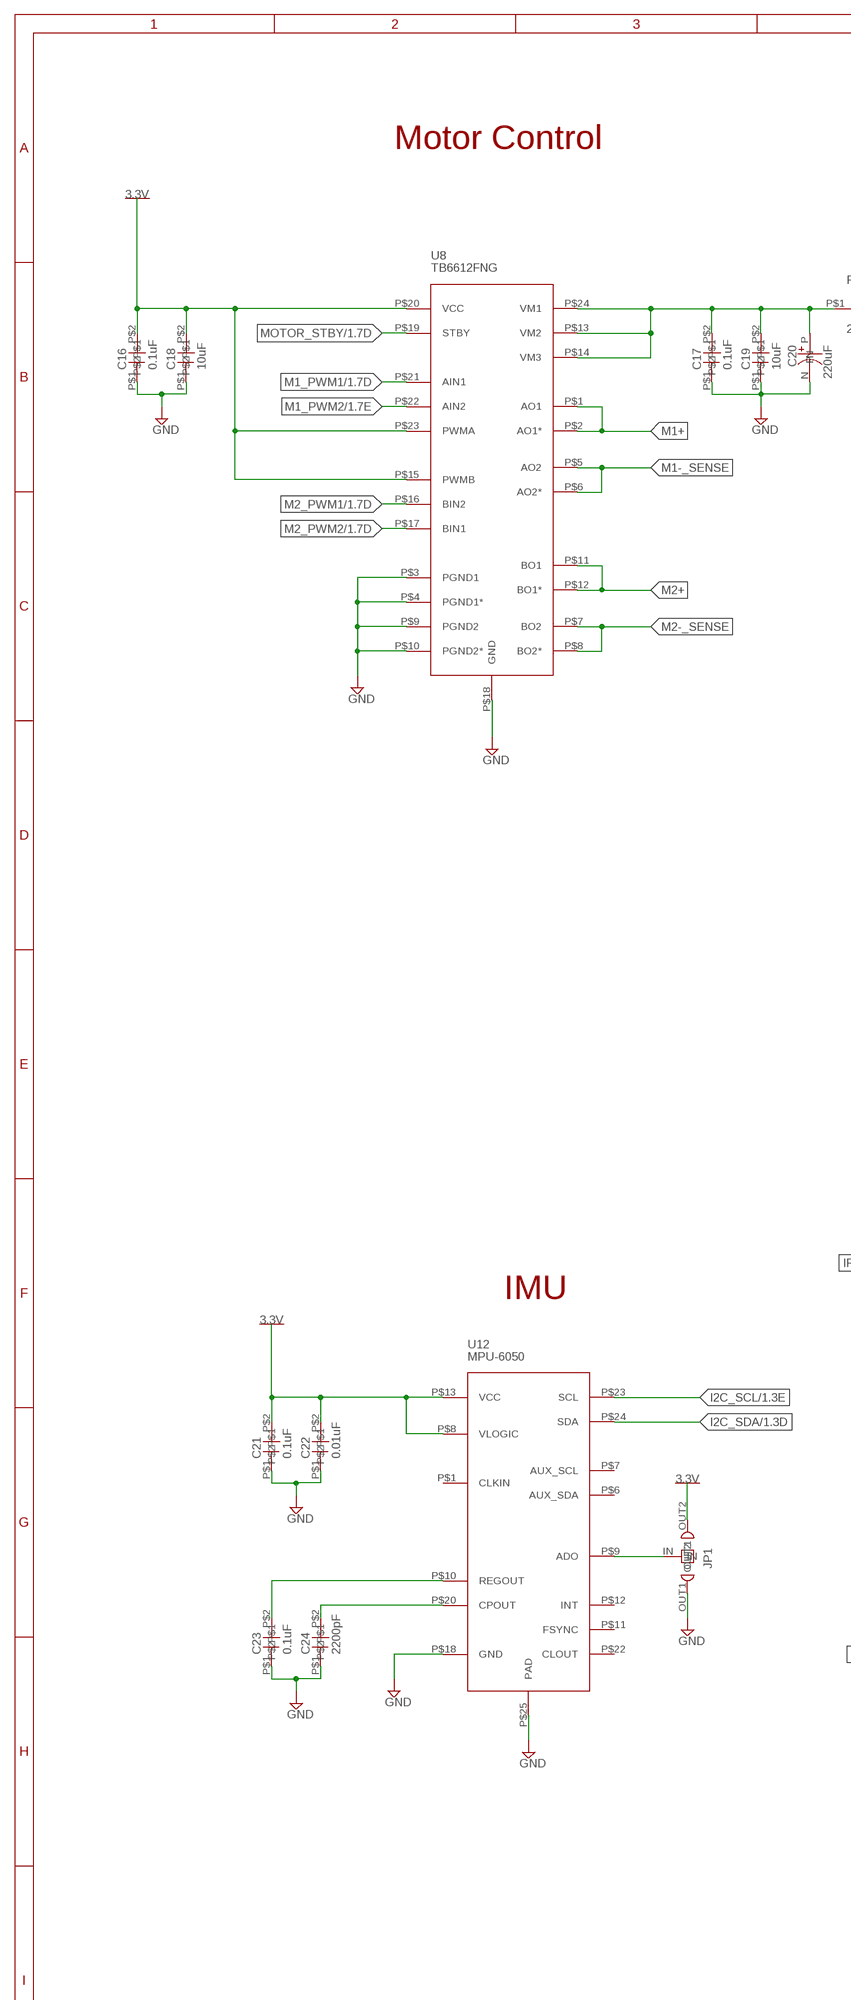
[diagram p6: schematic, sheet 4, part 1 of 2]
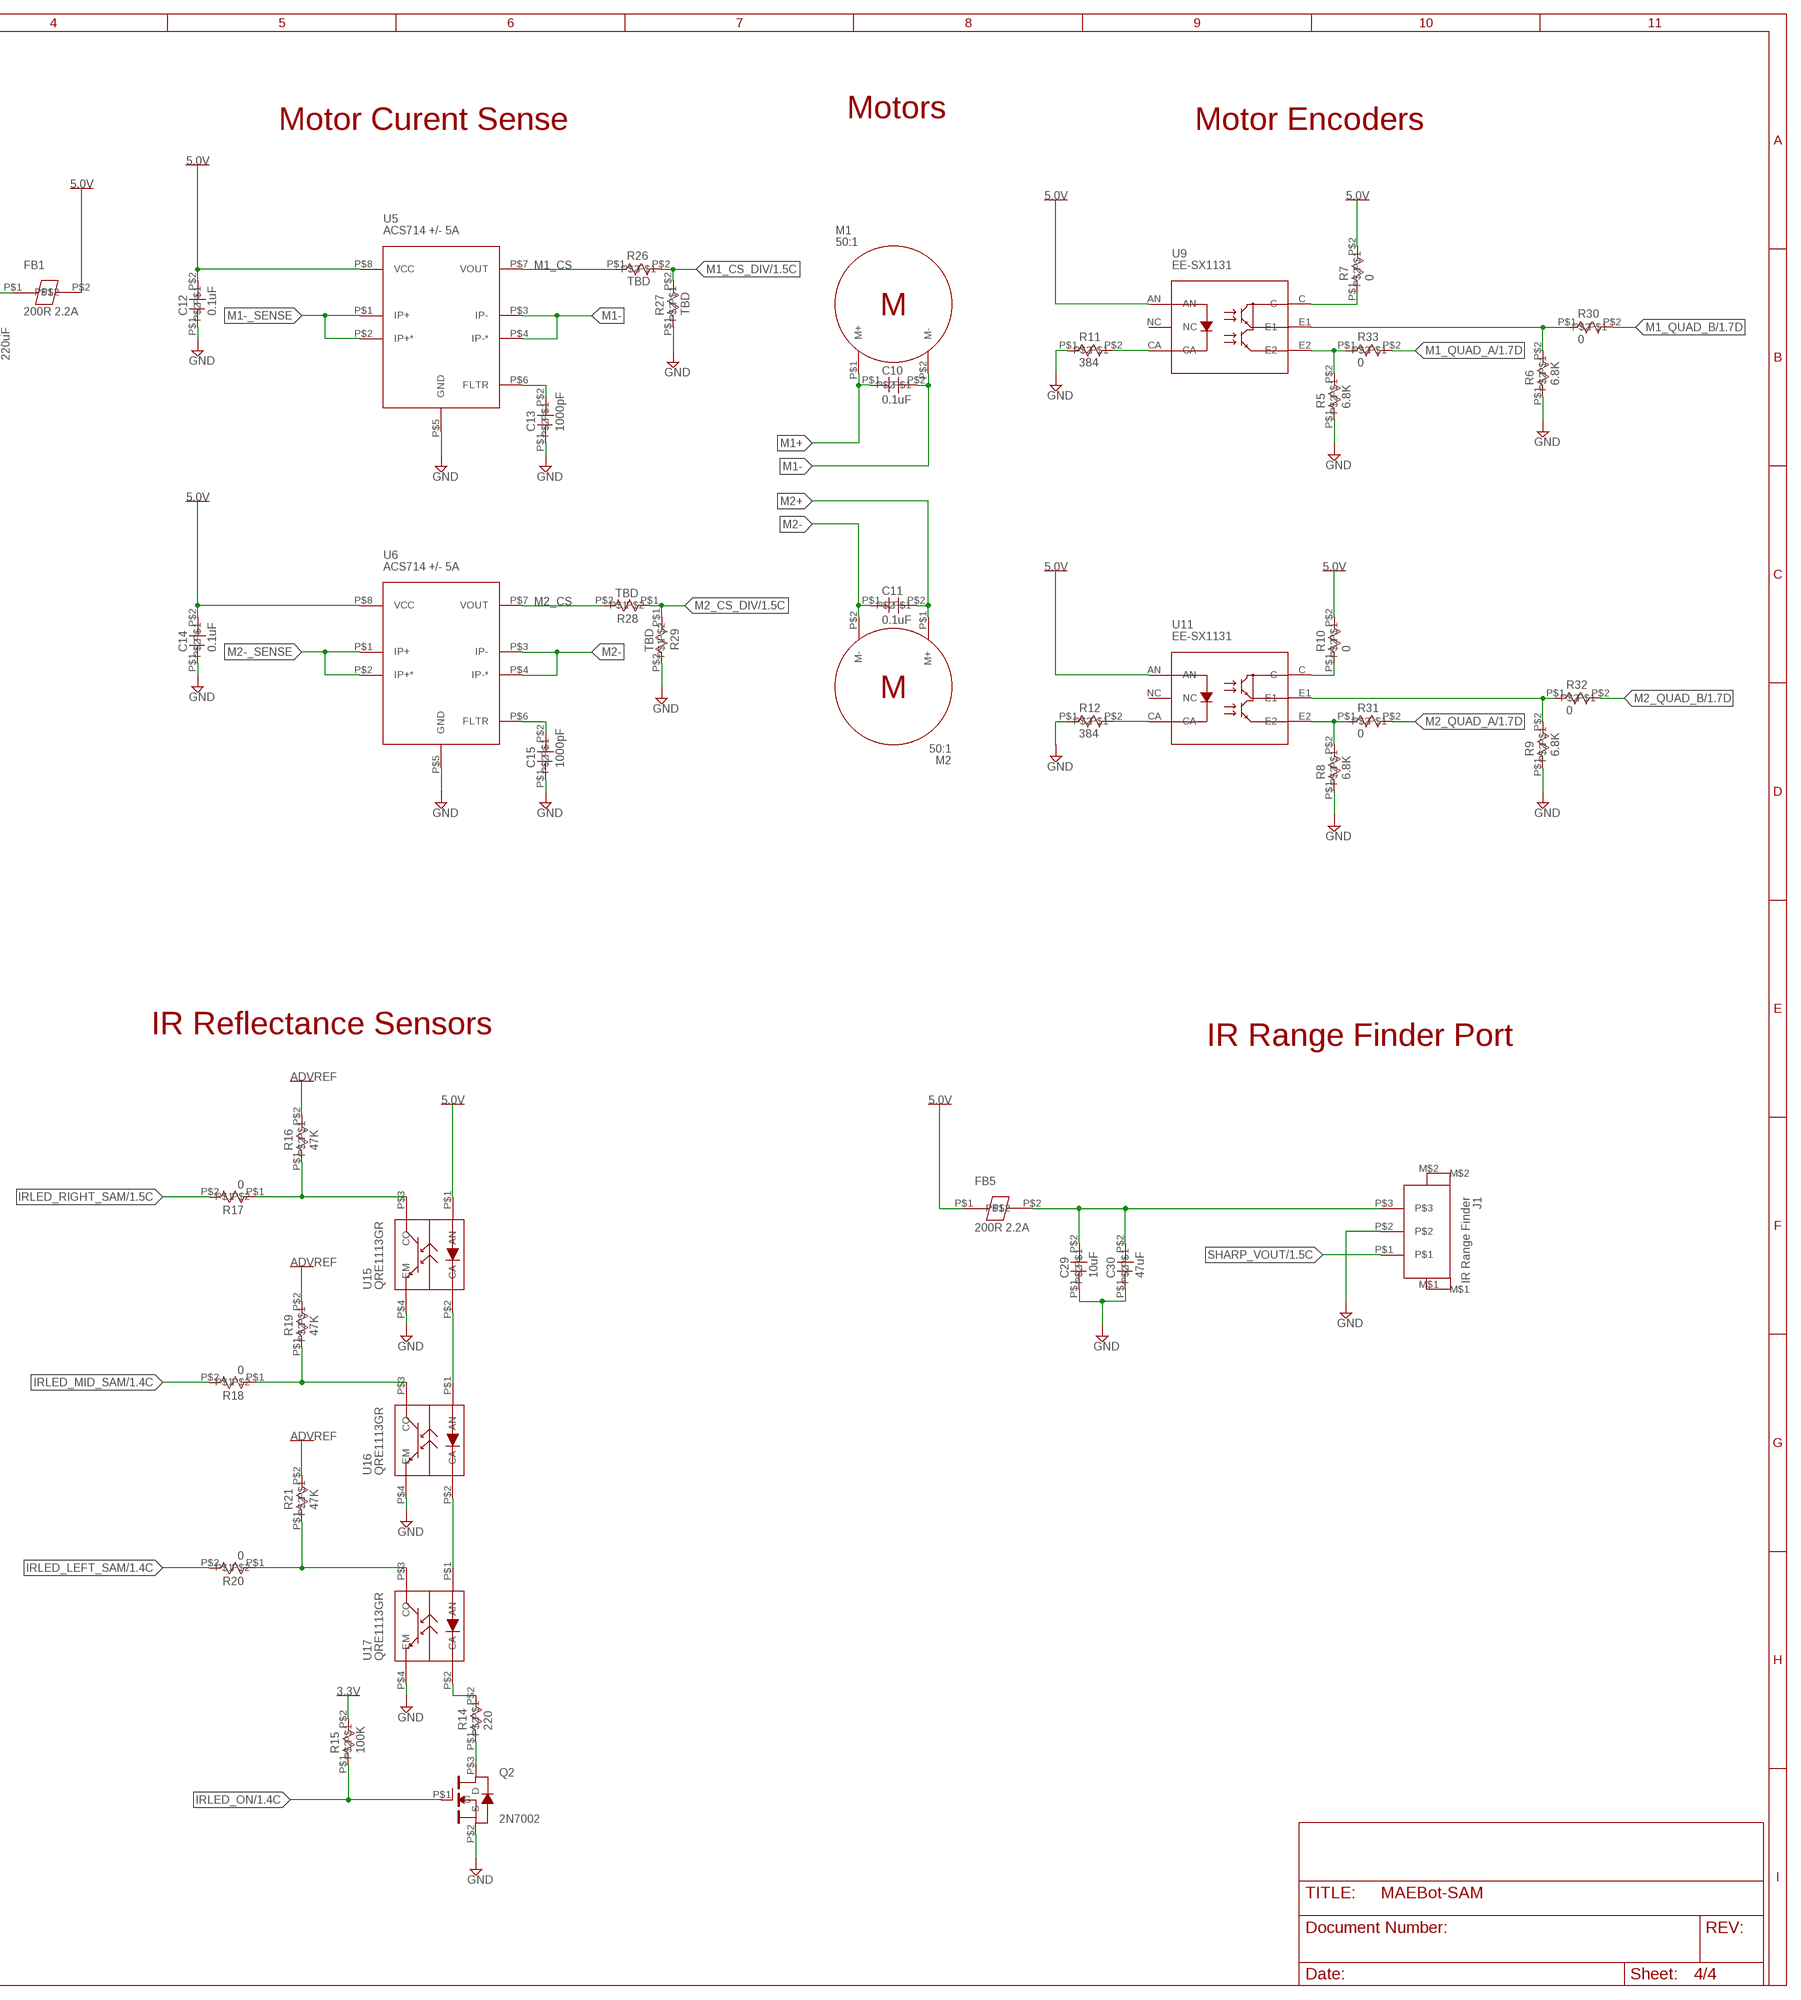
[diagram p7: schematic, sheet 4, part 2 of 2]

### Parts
C10  0.1uF  C0402  [R0402]
C11  0.1uF  C0402  [R0402]
C12  0.1uF  C0402  [R0402]
C13  1000pF  C0402  [R0402]
C14  0.1uF  C0402  [R0402]
C15  1000pF  C0402  [R0402]
C16  0.1uF  C0402  [R0402]
C17  0.1uF  C0402  [R0402]
C18  10uF  C0603  [SM0603]
C19  10uF  C0603  [SM0603]
C20  220uF  ECE-V1AA221XP  [VS_SERIES_D8]
C21  0.1uF  C0402  [R0402]
C22  0.01uF  C0402  [R0402]
C23  0.1uF  C0402  [R0402]
C24  2200pF  C0402  [R0402]
C29  10uF  C0603  [SM0603]
C30  47uF  C0805  [SM0805]
FB1  200R 2.2A  FB0603  [SM0603]
FB5  200R 2.2A  FB0603  [SM0603]
J1  IR Range Finder  PICOBLADE-3  [PICO-3]
JP1  JP0402  [JP0402]
M1  50:1  MMG_MOTOR  [MMG_MOTOR]
M2  50:1  MMG_MOTOR  [MMG_MOTOR]
Q2  2N7002  [SOT23]
R5  6.8K  R0402  [R0402]
R6  6.8K  R0402  [R0402]
R7  0  R0402  [R0402]
R8  6.8K  R0402  [R0402]
R9  6.8K  R0402  [R0402]
R10  0  R0402  [R0402]
R11  384  R0402  [R0402]
R12  384  R0402  [R0402]
R14  220  R0402  [R0402]
R15  100K  R0402  [R0402]
R16  47K  R0402  [R0402]
R17  0  R0402  [R0402]
R18  0  R0402  [R0402]
R19  47K  R0402  [R0402]
R20  0  R0402  [R0402]
R21  47K  R0402  [R0402]
R26  TBD  R0402  [R0402]
R27  TBD  R0402  [R0402]
R28  TBD  R0402  [R0402]
R29  TBD  R0402  [R0402]
R30  0  R0402  [R0402]
R31  0  R0402  [R0402]
R32  0  R0402  [R0402]
R33  0  R0402  [R0402]
U5  ACS714 +/- 5A  ACS714  [LC_8-PIN_SOIC]
U6  ACS714 +/- 5A  ACS714  [LC_8-PIN_SOIC]
U8  TB6612FNG  [SSOP24-P-300-0.65A]
U9  EE-SX1131  [EE-SX1131]
U11  EE-SX1131  [EE-SX1131]
U12  MPU-6050  [MPU-60X0]
U15  QRE1113GR  [QRE1113GR]
U16  QRE1113GR  [QRE1113GR]
U17  QRE1113GR  [QRE1113GR]

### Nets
3.3V: C16.P$2 C18.P$2 C21.P$2 C22.P$2 JP1.OUT2 R15.P$2 U8.P$15(PWMB) U8.P$20(VCC) U8.P$23(PWMA) U12.P$8(VLOGIC) U12.P$13(VCC) ; also sheet 1,2,3
5.0V: C12.P$2 C14.P$2 FB1.P$2 FB5.P$1 R7.P$2 R10.P$2 U5.P$8(VCC) U6.P$8(VCC) U9.AN U11.AN U15.P$1(AN) ; also sheet 2
ADVREF: R16.P$2 R19.P$2 R21.P$2 ; also sheet 1,2
CS_FLTR_1: C13.P$2 U5.P$6(FLTR)
CS_FLTR_2: C15.P$2 U6.P$6(FLTR)
GND: C12.P$1 C13.P$1 C14.P$1 C15.P$1 C16.P$1 C17.P$1 C18.P$1 C19.P$1 C20.N C21.P$1 C22.P$1 C23.P$1 C24.P$1 C29.P$1 C30.P$1 J1.P$2 JP1.OUT1 Q2.P$2(S) R5.P$1 R6.P$1 R8.P$1 R9.P$1 R11.P$1 R12.P$1 R27.P$1 R29.P$2 U5.P$5(GND) U6.P$5(GND) U8.P$3(PGND1) U8.P$4(PGND1*) U8.P$9(PGND2) U8.P$10(PGND2*) U8.P$18(GND) U12.P$18(GND) U12.P$25(PAD) U15.P$4(EM) U16.P$4(EM) U17.P$4(EM) ; also sheet 1,2,3
I2C_SCL: U12.P$23(SCL) ; also sheet 1
I2C_SDA: U12.P$24(SDA) ; also sheet 1
IRLED_LEFT: R20.P$1 R21.P$1 U17.P$3(CO)
IRLED_LEFT_SAM: R20.P$2 ; also sheet 1
IRLED_MID: R18.P$1 R19.P$1 U16.P$3(CO)
IRLED_MID_SAM: R18.P$2 ; also sheet 1
IRLED_ON: Q2.P$1(G) R15.P$1 ; also sheet 1
IRLED_RIGHT: R16.P$1 R17.P$1 U15.P$3(CO)
IRLED_RIGHT_SAM: R17.P$2 ; also sheet 1
M1+: C10.P$1 M1.P$1(M+) U8.P$1(AO1) U8.P$2(AO1*)
M1-: C10.P$2 M1.P$2(M-) U5.P$3(IP-) U5.P$4(IP-*)
M1-_SENSE: U5.P$1(IP+) U5.P$2(IP+*) U8.P$5(AO2) U8.P$6(AO2*)
M1_CS: R26.P$1 U5.P$7(VOUT)
M1_CS_DIV: R26.P$2 R27.P$2 ; also sheet 1
M1_E1: R6.P$2 R30.P$1 U9.E1
M1_E2: R5.P$2 R33.P$1 U9.E2
M1_PWM1: U8.P$21(AIN1) ; also sheet 1
M1_PWM2: U8.P$22(AIN2) ; also sheet 1
M1_QUAD_A: R33.P$2 ; also sheet 1
M1_QUAD_B: R30.P$2 ; also sheet 1
M2+: C11.P$2 M2.P$1(M+) U8.P$11(BO1) U8.P$12(BO1*)
M2-: C11.P$1 M2.P$2(M-) U6.P$3(IP-) U6.P$4(IP-*)
M2-_SENSE: U6.P$1(IP+) U6.P$2(IP+*) U8.P$7(BO2) U8.P$8(BO2*)
M2_CS: R28.P$2 U6.P$7(VOUT)
M2_CS_DIV: R28.P$1 R29.P$1 ; also sheet 1
M2_E1: R9.P$2 R32.P$1 U11.E1
M2_E2: R8.P$2 R31.P$1 U11.E2
M2_PWM1: U8.P$16(BIN2) ; also sheet 1
M2_PWM2: U8.P$17(BIN1) ; also sheet 1
M2_QUAD_A: R31.P$2 ; also sheet 1
M2_QUAD_B: R32.P$2 ; also sheet 1
MOTOR_STBY: U8.P$19(STBY) ; also sheet 1
MPU_AD: JP1.IN U12.P$9(ADO)
MPU_CP: C24.P$2 U12.P$20(CPOUT)
MPU_REG: C23.P$2 U12.P$10(REGOUT)
N$2: R7.P$1 U9.C
N$3: R12.P$2 U11.CA
N$6: U15.P$2(CA) U16.P$1(AN)
N$7: R11.P$2 U9.CA
N$8: U16.P$2(CA) U17.P$1(AN)
N$9: Q2.P$3(D) R14.P$1
N$10: R10.P$1 U11.C
N$13: R14.P$2 U17.P$2(CA)
SHARP_VOUT: J1.P$1 ; also sheet 1
V_MOT: C17.P$2 C19.P$2 C20.P FB1.P$1 U8.P$13(VM2) U8.P$14(VM3) U8.P$24(VM1)
V_SHARP: C29.P$2 C30.P$2 FB5.P$2 J1.P$3
Unconnected: J1.M$1 J1.M$2 U9.NC U11.NC U12.P$1(CLKIN) U12.P$6(AUX_SDA) U12.P$7(AUX_SCL) U12.P$11(FSYNC) U12.P$12(INT) U12.P$22(CLOUT)

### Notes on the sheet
- Motors
- Motor Curent Sense | Motor Encoders
- Motor Control
- IR Reflectance Sensors
- IR Range Finder Port
- IMU

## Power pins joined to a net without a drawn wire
VDD: U18.P$6(VDD)

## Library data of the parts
C1 C7-C17 C21-C25 C31 C32 C39 C53 C54 C56 C57 = res:C0402
C2 C3 C5 C6 C18 C19 C26 C27 C29 C40 C41 C43 C44 = res:C0603
C4 C30 C33 C42 C55 C58 = res:C0805
C20 = panasonic:ECE-V1AA221XP: Cap Aluminum
D1 D2 = vishay:SSA33L
D3-D7 D9 = res:LED0603
D10-D15 = res:TVS0603: Transient Voltage Supressor, SM0603
D16 D17 = res:TVS0402: Transient Voltage Supressor in an 0402 package
D25 D26 = res:DS0603: Schottky Diode SM0603
FB1-FB5 = res:FB0603
J1 = con-molex:PICOBLADE-3: 3-pin Picoblade
J2 = con-pinheader:J7X1: 7x1 0.100in pinheader
J3 J6 J7 = con-pinheader:J6X1: 6x1 0.100in pinheader
J4 = con-cui:PJ-002A-SMT: 2.0mm SURFACE MOUNT POWER JACK
J5 = con-molex:PICOBLADE-2: 2-pin Picoblade
J8 = con-molex:PICOBLADE-8: 8-pin Picoblade
JP1 = res:JP0402
L1 L2 = murata:VLF10040
M1 M2 = pololu:MMG_MOTOR: Micro Metal Gear Motor PCB Placement
PF1 = littlefuse:1210L: POLY-FUSE® Resettable PTC
Q1 Q2 = trans:2N7002: N-Channel MOSFET
R1-R37 = res:R0402: Resistor, Surface Mount, 0402
SAMA1 = april:SAMA5_CARRIER
SB1 SB2 = res:SB0402: Solder Bridge, Surface Mount, 0402
SW1 = te:FSMJSMA: Tactile Switch OFF-MOM, Surface Mount
U1 = analog-devices:ADP2303ADRZ-3.3-R7: 2A/3A, 20V to 3.3V, 700kHz Nonsynchronous Step-Down Regulator
U2 = micrel:MIC2788: Push-button Reset IC
U3 = maxim:MAX6816: CMOS Switch Debouncer with ±15kV ESD Protection
U4 = maxim:MAX16045: On/Off Controller with Debounce and ±15kV ESD Protection
U5 U6 = allegro:ACS714: Hall Effect-Based Linear Current Sensor IC
U7 U14 = texas:LP2985
U8 = toshiba:TB6612FNG: Driver IC for Dual DC motor
U9 U11 = omron:EE-SX1131: Photo Microsensor
U10 = analog-devices:ADP2303ADRZ-5.0-R7
U12 = invensense:MPU-6050: IMU
U13 = analog-devices:ADP1713: 300 mA, Low Dropout CMOS Linear Regulator
U15-U17 = fairchild:QRE1113GR: SMT Reflective Object Sensor
U18 = sillabs:CP2102: USB to UART Converter
USB1 = con-jae:USB_MINI_A
USB2 = omron:XM7A-0442-A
